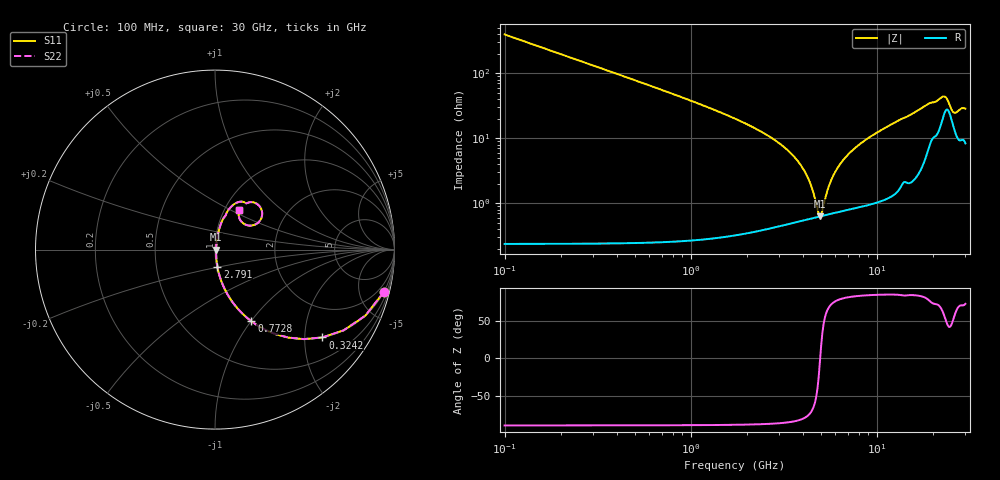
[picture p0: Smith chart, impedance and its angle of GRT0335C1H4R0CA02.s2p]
!Murata Part Number: GRT0335C1H4R0CA02
!These Parameters are Measured in Series Mode Connection
!Data Generated on Jun 19, 2026
!  o--ll--o
!Port1  Port2
!  o------o
!Operation Temp=25[degC], DC Bias Voltage=0[V]
!Freq. Start=100[MHz] Stop=30[GHz] 401[Steps]
# Hz S RI R 50
!Freq.(Hz) S11(Real) S11(Imag) S21(Real) S21(Imag) S12(Real) S12(Imag) S22(Real) S22(Imag)
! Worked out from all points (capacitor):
!   401 points, 100 MHz to 30 GHz, reference 50 ohm
!   read as one part in series: C = 4 pF near 249.5 MHz
!   lowest |Z| = 629 mohm at 4.959 GHz (marker M1)
!   series resonance near 4.97 GHz, so ESL is about 260 pH
!   S11 on the Smith chart (normalised r, x): 100 MHz: 1.00, -7.95; 324.2 MHz: 1.00, -2.44; 772.8 MHz: 1.01, -1.00; 2.791 GHz: 1.01, -0.19; 30 GHz: 1.17, +0.55
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1e8  0.9404 -0.2364  0.0596 0.2364  0.0596 0.2364  0.9404 -0.2364
3.2425e8  0.5986 -0.4892  0.4014 0.4892  0.4014 0.4892  0.5986 -0.4892
5.485e8  0.3396 -0.4719  0.6604 0.4719  0.6604 0.4719  0.3396 -0.4719
7.7275e8  0.2025 -0.3993  0.7975 0.3993  0.7975 0.3993  0.2025 -0.3993
1.4455e9  0.0618 -0.235  0.9382 0.235  0.9382 0.235  0.0618 -0.235
2.791e9  0.0133 -0.0951  0.9867 0.0951  0.9867 0.0951  0.0133 -0.0951
4.06175e9  0.00645 -0.0317  0.9936 0.0317  0.9936 0.0317  0.00645 -0.0317
4.4355e9  0.0061 -0.0178  0.9939 0.0178  0.9939 0.0178  0.0061 -0.0178
4.80925e9  0.00614 -0.00513  0.9939 0.00513  0.9939 0.00513  0.00614 -0.00513
4.95875e9  0.00624 -0.000356  0.9938 0.000356  0.9938 0.000356  0.00624 -0.000356
5.10825e9  0.00638 0.00427  0.9936 -0.00427  0.9936 -0.00427  0.00638 0.00427
5.40725e9  0.00678 0.0131  0.9932 -0.0131  0.9932 -0.0131  0.00678 0.0131
5.70625e9  0.00732 0.0215  0.9927 -0.0215  0.9927 -0.0215  0.00732 0.0215
6.60325e9  0.00954 0.0447  0.9905 -0.0447  0.9905 -0.0447  0.00954 0.0447
8.0235e9  0.0146 0.077  0.9854 -0.077  0.9854 -0.077  0.0146 0.077
1.01165e10  0.0248 0.1194  0.9752 -0.1194  0.9752 -0.1194  0.0248 0.1194
1.505e10  0.0658 0.2067  0.9342 -0.2067  0.9342 -0.2067  0.0658 0.2067
2.005825e10  0.1717 0.2585  0.8283 -0.2585  0.8283 -0.2585  0.1717 0.2585
2.304825e10  0.2582 0.2246  0.7418 -0.2246  0.7418 -0.2246  0.2582 0.2246
2.50665e10  0.1959 0.1336  0.8041 -0.1336  0.8041 -0.1336  0.1959 0.1336
2.618775e10  0.1471 0.1558  0.8529 -0.1558  0.8529 -0.1558  0.1471 0.1558
3e10  0.1329 0.2201  0.8671 -0.2201  0.8671 -0.2201  0.1329 0.2201
